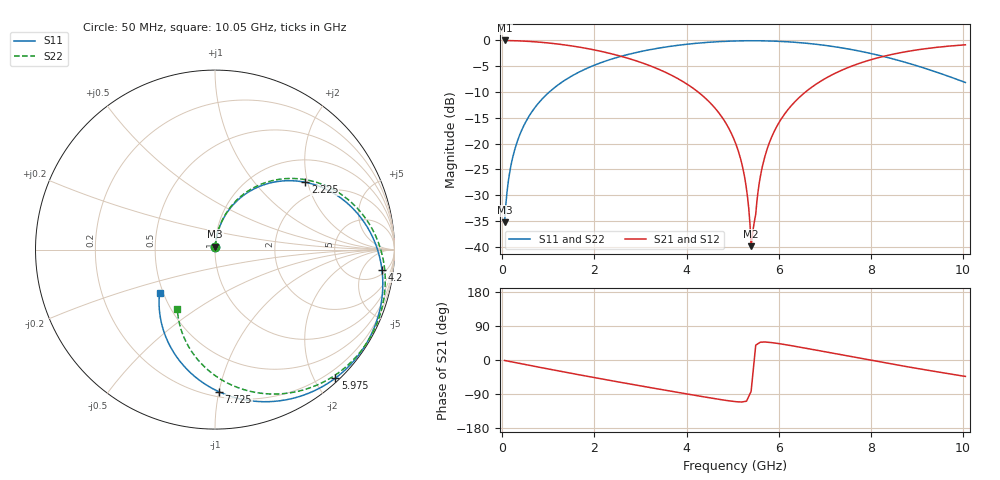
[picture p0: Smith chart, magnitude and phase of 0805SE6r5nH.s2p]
! AVX Thin Film Operation		Date: May 2002
! Description: Accu-L® Series, Thin Film, SMD, RF Inductors
! Part Number: L08056R5CEWTR
! 50 MHz  -  10.05 GHz
! Serial Measurements
# mhz S db R 50
!	S11		S21		S12		S22
!	dB	Phase	dB	Phase	dB	Phase	dB	Phase
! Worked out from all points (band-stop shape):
!   401 points, 50 MHz to 10.05 GHz, reference 50 ohm
!   highest |S21| = -0.01 dB at 50 MHz (marker M1); lowest = -39.9 dB at 5.4 GHz (marker M2)
!   |S21| within 3 dB of the highest: start of sweep to 2.549 GHz; 8.31 GHz to end of sweep
!   lowest |S11| = -35.3 dB at 50 MHz (marker M3), VSWR 1.04, Z = 50.1 + j1.72 ohm
!   |S11| at or under -10 dB: start of sweep to 1.02 GHz
!   |S22| runs from -35.3 to -0.1 dB; largest |S21 - S12| = 0
!   S11 on the Smith chart (normalised r, x): 50 MHz: 1.00, +0.03; 2.225 GHz: 1.56, +1.94; 4.2 GHz: 7, -13; 5.975 GHz: 0.06, -2.30; 7.725 GHz: 0.23, -1.00; 10.05 GHz: 0.48, -0.27
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50  -35.28 85.7  -0.01 -1.3  -0.01 -1.3  -35.28 85.7
150  -26.14 83.9  -0.03 -3.7  -0.03 -3.7  -26.14 84.0
225  -22.70 82.4  -0.05 -5.5  -0.05 -5.5  -22.70 82.6
525  -15.52 75.8  -0.16 -12.6  -0.16 -12.6  -15.52 76.2
1025  -9.96 64.2  -0.52 -24.3  -0.52 -24.3  -9.96 65.0
1725  -5.87 48.0  -1.39 -40.3  -1.39 -40.3  -5.87 49.5
2225  -4.05 36.7  -2.28 -51.4  -2.28 -51.4  -4.05 38.6
3400  -1.48 10.7  -5.62 -76.8  -5.62 -76.8  -1.48 13.7
4200  -0.57 -6.8  -9.66 -93.6  -9.66 -93.6  -0.56 -3.0
4700  -0.24 -17.9  -14.04 -103.7  -14.04 -103.7  -0.24 -13.4
5050  -0.11 -25.7  -19.64 -109.7  -19.64 -109.7  -0.11 -20.8
5250  -0.07 -30.2  -26.06 -109.8  -26.06 -109.8  -0.07 -25.1
5400  -0.06 -33.7  -39.87 -82.6  -39.87 -82.6  -0.06 -28.3
5450  -0.06 -34.8  -36.23 -21.7  -36.23 -21.7  -0.06 -29.4
5575  -0.07 -37.7  -27.73 45.0  -27.73 45.0  -0.07 -32.1
5675  -0.08 -40.0  -23.27 47.4  -23.27 47.4  -0.08 -34.2
5975  -0.17 -46.9  -16.38 43.7  -16.38 43.7  -0.16 -40.7
6725  -0.66 -64.6  -9.00 28.0  -9.00 28.0  -0.66 -57.1
7725  -2.02 -88.4  -4.52 5.5  -4.52 5.5  -2.01 -78.8
8400  -3.40 -104.3  -2.82 -9.4  -2.82 -9.4  -3.38 -92.7
9200  -5.49 -122.8  -1.58 -26.4  -1.58 -26.4  -5.46 -108.0
10050  -8.15 -142.1  -0.85 -43.3  -0.85 -43.3  -8.10 -122.2
